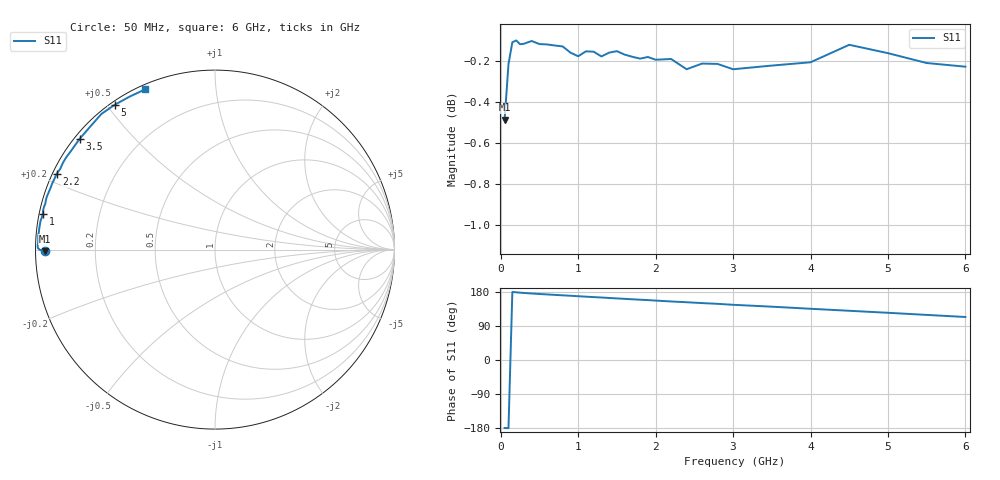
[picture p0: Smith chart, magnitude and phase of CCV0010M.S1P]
! Infineon Technologies  Discrete & RF Semiconductors
! BBY57-02W
! Si Tuning Diode in SCD-80
! VR = 0
! S-Parameters:  June  2000
# GHz  S  MA  R  50
!  f  S11
! GHz  MAG  ANG
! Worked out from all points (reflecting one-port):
!   34 points, 50 MHz to 6 GHz, reference 50 ohm
!   lowest |S11| = -0.5 dB at 50 MHz (marker M1), VSWR 35.70, Z = 1.4 - j0.218 ohm
!   phase of S11 starts at -180 deg and turns -67 deg over the sweep
!   S11 on the Smith chart (normalised r, x): 50 MHz: 0.03, -0.00; 1 GHz: 0.01, +0.10; 2.2 GHz: 0.01, +0.23; 3.5 GHz: 0.01, +0.36; 5 GHz: 0.01, +0.52; 6 GHz: 0.02, +0.66
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0.05  0.9455 -179.5
0.1  0.9753 -179.9
0.15  0.9873 179.5
0.2  0.9883 178.6
0.25  0.9862 177.7
0.4  0.988 175.5
0.6  0.9861 173.0
0.8  0.985 170.7
0.9  0.9816 169.6
1  0.9796 168.3
1.1  0.9823 167.1
1.2  0.9821 166.0
1.3  0.9795 164.9
1.5  0.9824 162.5
1.6  0.9805 161.4
1.8  0.9783 159.1
1.9  0.9792 158.1
2.2  0.9781 154.5
2.4  0.9725 152.4
2.6  0.9756 150.2
2.8  0.9754 148.2
3  0.9725 145.7
3.5  0.9745 140.7
4  0.9763 135.2
4.5  0.9859 129.9
5  0.9813 124.6
5.5  0.9759 119.0
6  0.9739 113.5
